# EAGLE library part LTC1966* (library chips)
Precision Micropower, DS RMS-to-DC Converter
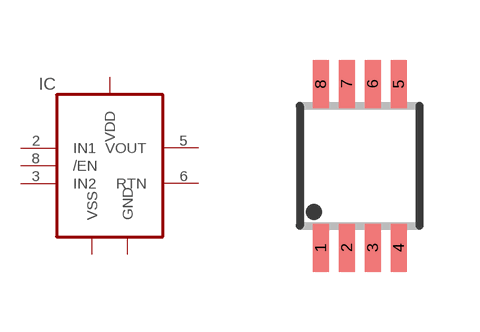
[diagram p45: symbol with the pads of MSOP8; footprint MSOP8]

Designator prefix IC

## LTC1966CMS8, LTC1966IMS8  [MSOP8]
1  GND
2  IN1  in
3  IN2  in
4  VSS
5  VOUT  out
6  RTN  pas
7  VDD
8  /EN  in

## Footprint MSOP8 (pad centres in mm)
MSOP8
smd 0.4 x 1.2: 1 -0.975,-2.05; 2 -0.325,-2.05; 3 0.325,-2.05; 4 0.975,-2.05; 5 0.975,2.05; 6 0.325,2.05; 7 -0.325,2.05; 8 -0.975,2.05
